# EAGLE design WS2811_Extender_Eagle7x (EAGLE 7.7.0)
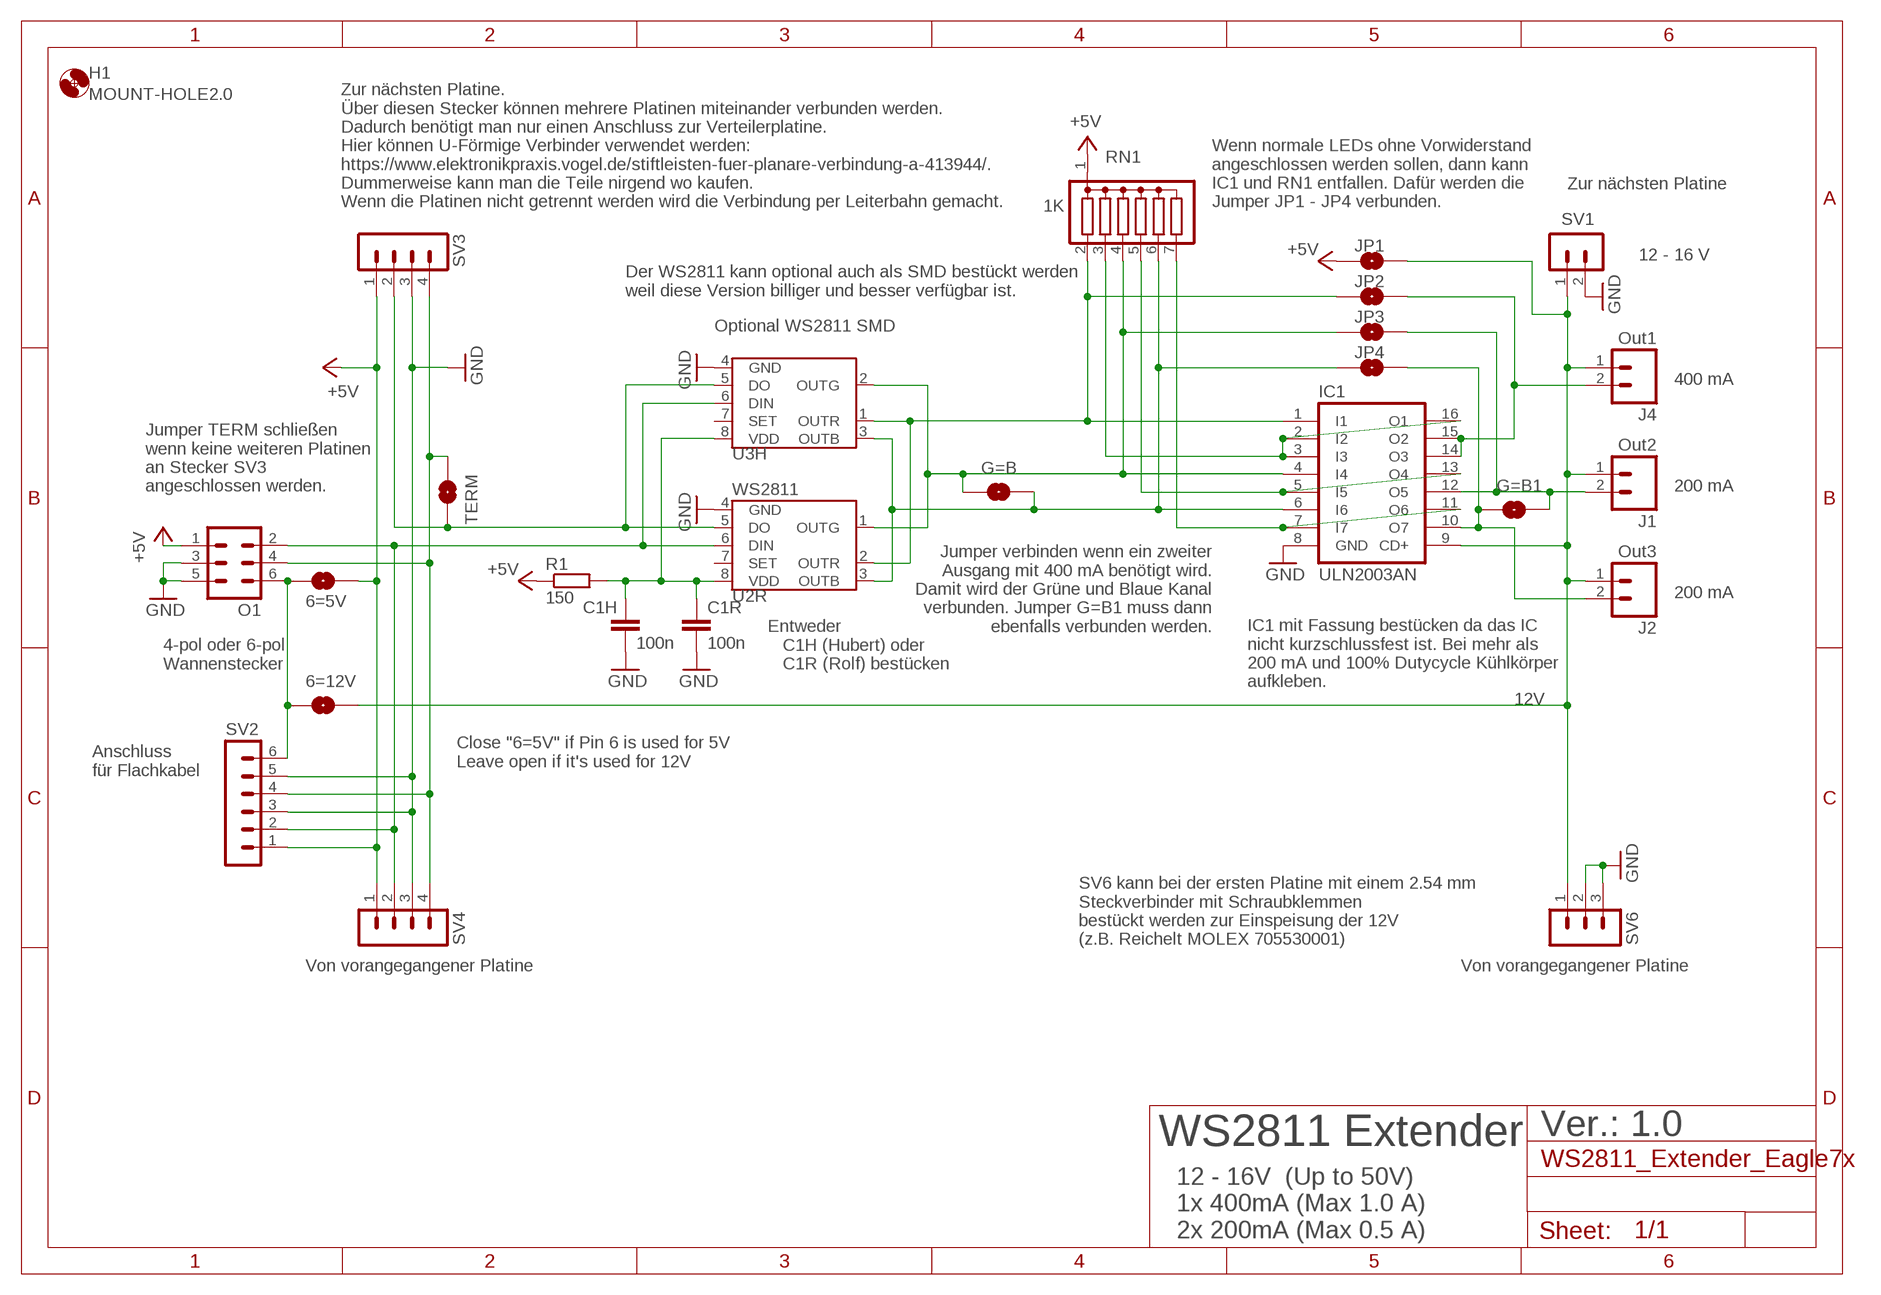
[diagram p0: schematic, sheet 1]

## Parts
6=5V  SOLDERJUMPERNO  [SJ_2S-NO]
6=12V  SOLDERJUMPERNO  [SJ_2S-NO]
C1H  100n  C-EUC1206  [C1206]
C1R  100n  C-EU025-024X044  [C025-024X044]
G=B  SOLDERJUMPERNO  [SJ_2S-NO]
G=B1  SOLDERJUMPERNO  [SJ_2S-NO]
H1  MOUNT-HOLE2.0  [2,0]
IC1  ULN2003AN  [DIL16]
J1  Out2  M02PTH  [1X02]
J2  Out3  M02PTH  [1X02]
J4  Out1  M02PTH  [1X02]
JP1  SOLDERJUMPERNO  [SJ_2S-NO]
JP2  SOLDERJUMPERNO  [SJ_2S-NO]
JP3  SOLDERJUMPERNO  [SJ_2S-NO]
JP4  SOLDERJUMPERNO  [SJ_2S-NO]
O1  ML6  [ML6]
R1  150  RCL_R-EU_0207/2V  [RCL_0207/2V]
RN1  1K  G06R  [SIL7]
SV1  MA02-1  [MA02-1]
SV2  MA06-1  [MA06-1]
SV3  MA04-1  [MA04-1]
SV4  MA04-1  [MA04-1]
SV6  MA03-1  [MA03-1]
TERM  SOLDERJUMPERNO  [SJ_2S-NO]
U2R  WS2811  S3PO_MODUL_WS2811_SOUND_MP3-TF-16P_WS2811_AND_ATTINY_WS2811-ICTINY45-20-DIP  [S3PO_MODUL_WS2811_SOUND_MP3-TF-16P_WS2811_AND_ATTINY_WS2811_DIP08]
U3H  WS2811 SOT-8  S3PO_MODUL_WS2811_SOUND_MP3-TF-16P_WS2811_AND_ATTINY_WS2811-ICSOP8  [SOP8]

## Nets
12V: 6=12V.2 IC1.9(CD+) J1.1 J2.1 J4.1 JP1.2 SV1.1 SV6.1
+5V: 6=5V.2 JP1.1 O1.1 R1.1 RN1.1 SV2.1 SV3.1 SV4.1
GND: C1H.2 C1R.2 IC1.8(GND) O1.3 O1.5 SV1.2 SV2.3 SV2.5 SV3.3 SV4.3 SV6.2 SV6.3 U2R.4(GND) U3H.4(GND)
N$1: O1.2 SV2.2 SV4.2 U2R.6(DIN) U3H.6(DIN)
N$2: SV3.2 TERM.2 U2R.5(DO) U3H.5(DO)
N$3: O1.4 SV2.4 SV3.4 SV4.4 TERM.1
N$4: C1H.1 C1R.1 R1.2 U2R.8(VDD) U3H.8(VDD)
N$5: IC1.1(I1) JP2.1 RN1.2 U2R.2(OUTR) U3H.1(OUTR)
N$6: 6=5V.1 6=12V.1 O1.6 SV2.6
N$8: G=B.2 IC1.6(I6) JP4.1 RN1.6 U2R.3(OUTB) U3H.3(OUTB)
N$9: IC1.2(I2) IC1.3(I3) IC1.16(O1) RN1.3
N$11: IC1.5(I5) IC1.13(O4) RN1.5
N$12: IC1.7(I7) IC1.11(O6) RN1.7
N$21: G=B.1 IC1.4(I4) JP3.1 RN1.4 U2R.1(OUTG) U3H.2(OUTG)
O1: IC1.14(O3) IC1.15(O2) J4.2 JP2.2
O2: G=B1.2 IC1.12(O5) J1.2 JP3.2
O3: G=B1.1 IC1.10(O7) J2.2 JP4.2
Unconnected: U2R.7(SET) U3H.7(SET)

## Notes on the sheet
- Zur nächsten Platine
- Zur nächsten Platine. 
  Über diesen Stecker können mehrere Platinen miteinander verbunden werden.
  Dadurch benötigt man nur einen Anschluss zur Verteilerplatine.
  Hier können U-Förmige Verbinder verwendet werden: 
  https://www.elektronikpraxis.vogel.de/stiftleisten-fuer-planare-verbindung-a-413944/.
  Dummerweise kann man die Teile nirgend wo kaufen.
  Wenn die Platinen nicht getrennt werden wird die Verbindung per Leiterbahn gemacht.
- Wenn normale LEDs ohne Vorwiderstand
  angeschlossen werden sollen, dann kann
  IC1 und RN1 entfallen. Dafür werden die
  Jumper JP1 - JP4 verbunden.
- 12 - 16 V
- Der WS2811 kann optional auch als SMD bestückt werden
  weil diese Version billiger und besser verfügbar ist.
- Optional WS2811 SMD
- 400 mA
- Jumper TERM schließen 
  wenn keine weiteren Platinen
  an Stecker SV3 
  angeschlossen werden.
- 200 mA
- Jumper verbinden wenn ein zweiter
  Ausgang mit 400 mA benötigt wird.
  Damit wird der Grüne und Blaue Kanal
  verbunden. Jumper G=B1 muss dann
  ebenfalls verbunden werden.
- 200 mA
- 4-pol oder 6-pol 
  Wannenstecker
- Entweder 
     C1H (Hubert) oder 
     C1R (Rolf) bestücken
- IC1 mit Fassung bestücken da das IC
  nicht kurzschlussfest ist. Bei mehr als 
  200 mA und 100% Dutycycle Kühlkörper
  aufkleben.
- Close "6=5V" if Pin 6 is used for 5V
  Leave open if it's used for 12V
- Anschluss
  für Flachkabel
- SV6 kann bei der ersten Platine mit einem 2.54 mm
  Steckverbinder mit Schraubklemmen
  bestückt werden zur Einspeisung der 12V
  (z.B. Reichelt MOLEX 705530001)
- Von vorangegangener Platine | Von vorangegangener Platine
- WS2811 Extender | Ver.: 1.0
- 12 - 16V  (Up to 50V)
  1x 400mA (Max 1.0 A)
  2x 200mA (Max 0.5 A)

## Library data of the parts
6=5V 6=12V G=B G=B1 JP1-JP4 TERM = SparkFun-Retired:SOLDERJUMPER: Solder Jumper
C1H C1R = rcl:C-EU: CAPACITOR, European symbol; SPICEPREFIX: C
H1 = holes:MOUNT-HOLE: MOUNTING HOLE with drill center marker
IC1 = uln-udn:ULN2003A: DRIVER ARRAY; REICHELT: ULN 2003A STM; REICHELT_EU: 0,22 €; REICHELT_LNK: https://www.reichelt.de/seven-darlington-arrays-dip-16-uln-2003a-stm-p216685.html?&trstct=pos_0
J1 J2 J4 = SparkFun-Connectors:M02: Standard 2-pin 0.1" header. Use with
O1 = con-harting-ml:ML6: HARTING; OC_FARNELL: unknown; OC_NEWARK: unknown
R1 = Sound_MP3-TF-16P_and_WS2811:RCL_R-EU_: RESISTOR, European symbol; SPICEPREFIX: R
RN1 = resistor-sil:G06R: SIL RESISTOR; OC_FARNELL: unknown; OC_NEWARK: unknown; REICHELT: SIL 7-6 1,0K; REICHELT_EU: 0,071 €; REICHELT_LNK: https://www.reichelt.de/widerstandsnetzwerk-1-0-kohm-sternschaltung-6wid-7pins-sil-7-6-1-0k-p17841.html?&trstct=pol_1
SV1 = con-lstb:MA02-1: PIN HEADER
SV2 = con-lstb:MA06-1: PIN HEADER; OC_FARNELL: unknown; OC_NEWARK: unknown
SV3 SV4 = con-lstb:MA04-1: PIN HEADER
SV6 = con-lstb:MA03-1: PIN HEADER
U2R = S3PO_Modul_WS2811:S3PO_MODUL_WS2811_SOUND_MP3-TF-16P_WS2811_AND_ATTINY_WS2811-IC: Die Pin nummern im Dokument https://cdn-shop.adafruit.com/datasheets/WS2811.pdf für R und G sind vertauscht ;-(; PROD_ID: IC-09439; VALUE: TINY45-20-DIP
U3H = S3PO_Modul_WS2811:S3PO_MODUL_WS2811_SOUND_MP3-TF-16P_WS2811_AND_ATTINY_WS2811-IC: Die Pin nummern im Dokument https://cdn-shop.adafruit.com/datasheets/WS2811.pdf für R und G sind vertauscht ;-(

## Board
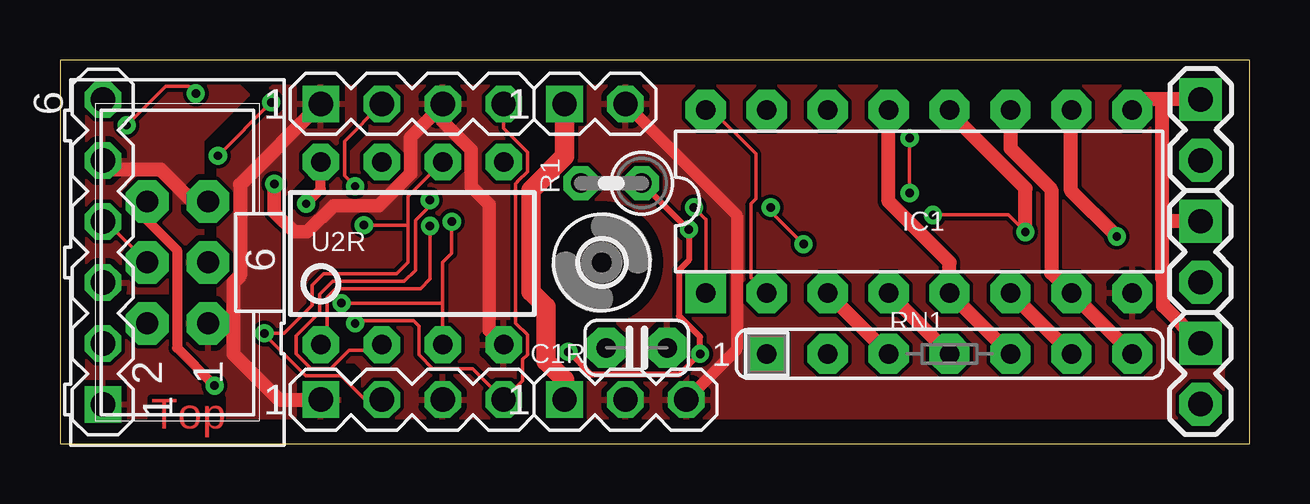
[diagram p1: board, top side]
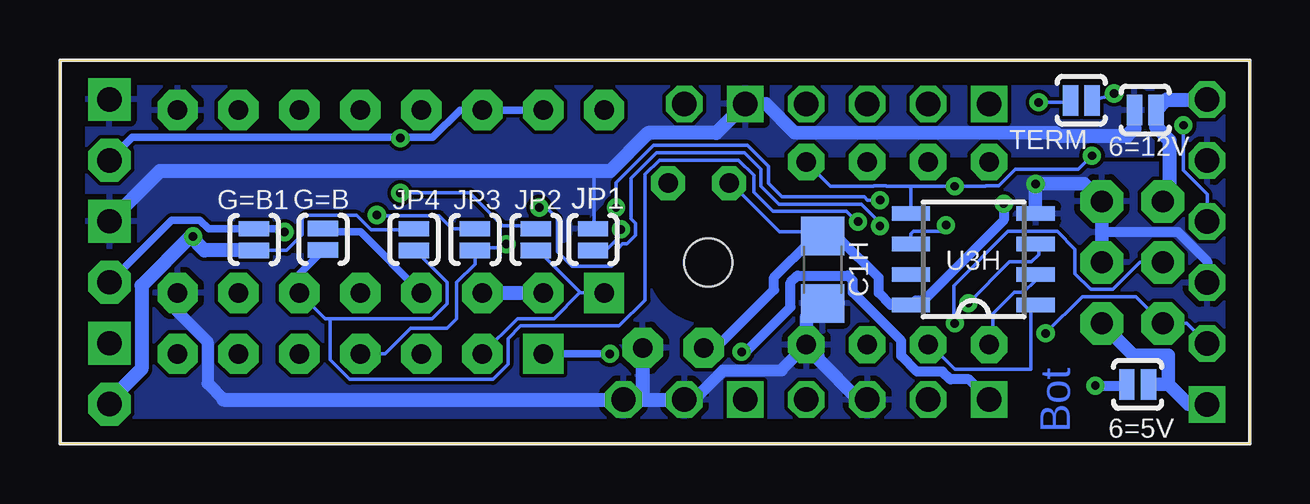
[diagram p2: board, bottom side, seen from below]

Size 49.6 x 15.99 mm. Coordinates in mm from the lower left corner, seen from the top.
Outline: 0,0 49.6,0 49.6,15.99 0,15.99 0,0
Copper layers (1*16): Top 0.035mm / dielectric 1.5mm / Bottom 0.035mm
Design rules "default": minimum track width 6mil, minimum drill 0.35mm, track to track 6mil, track to pad 6mil, pad to pad 6mil, via to via 6mil, smd to smd 6mil, copper to edge 40mil, drill to drill 6mil, minimum pad ring 10mil, minimum via ring 8mil, stop-mask expansion 4mil, vias tented up to drill 0mil, thermal gap 10mil

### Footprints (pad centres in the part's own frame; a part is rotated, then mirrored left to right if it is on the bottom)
SJ_2S-NO = smd 0.635 x 1.27: 1 -0.45,0; 2 0.45,0
C1206 = smd 1.6 x 1.8: 1 -1.4,0; 2 1.4,0
C025-024X044 = drill 0.813 pad 1.676 octagon: 1 -1.27,0; 2 1.27,0
2,0 = hole 2: 0,0
DIL16 = drill 0.813 pad 1.676 square: 1 -8.89,-3.81 | drill 0.813 pad 1.676 octagon: 2 -6.35,-3.81; 3 -3.81,-3.81; 4 -1.27,-3.81; 5 1.27,-3.81; 6 3.81,-3.81; 7 6.35,-3.81; 8 8.89,-3.81; 9 8.89,3.81; 10 6.35,3.81; 11 3.81,3.81; 12 1.27,3.81; 13 -1.27,3.81; 14 -3.81,3.81; 15 -6.35,3.81; 16 -8.89,3.81
1X02 = drill 1.016 pad 1.778 square: 1 0,0 | drill 1.016 pad 1.778 octagon: 2 2.54,0
ML6 = drill 0.914 pad 1.778 octagon: 1 -2.54,-1.27; 2 -2.54,1.27; 3 0,-1.27; 4 0,1.27; 5 2.54,-1.27; 6 2.54,1.27
RCL_0207/2V = drill 0.813 pad 1.422 octagon: 1 -1.27,0; 2 1.27,0
SIL7 = drill 0.813 pad 1.676 square: 1 -7.62,0 | drill 0.813 pad 1.676 octagon: 2 -5.08,0; 3 -2.54,0; 4 0,0; 5 2.54,0; 6 5.08,0; 7 7.62,0
MA02-1 = drill 1.016 pad 1.524 square: 1 -1.27,0 | drill 1.016 pad 1.524 octagon: 2 1.27,0
MA06-1 = drill 1.016 pad 1.524 square: 1 -6.35,0 | drill 1.016 pad 1.524 octagon: 2 -3.81,0; 3 -1.27,0; 4 1.27,0; 5 3.81,0; 6 6.35,0
MA04-1 = drill 1.016 pad 1.524 square: 1 -3.81,0 | drill 1.016 pad 1.524 octagon: 2 -1.27,0; 3 1.27,0; 4 3.81,0
MA03-1 = drill 1.016 pad 1.524 square: 1 -3.81,0 | drill 1.016 pad 1.524 octagon: 2 -1.27,0; 3 1.27,0
S3PO_MODUL_WS2811_SOUND_MP3-TF-16P_WS2811_AND_ATTINY_WS2811_DIP08 = drill 0.813 pad 1.524 octagon: 1 -3.81,-3.81; 2 -1.27,-3.81; 3 1.27,-3.81; 4 3.81,-3.81; 5 3.81,3.81; 6 1.27,3.81; 7 -1.27,3.81; 8 -3.81,3.81
SOP8 = smd 0.6 x 1.6: 1 -1.905,-2.6; 2 -0.635,-2.6; 3 0.635,-2.6; 4 1.905,-2.6; 5 1.905,2.6; 6 0.635,2.6; 7 -0.635,2.6; 8 -1.905,2.6

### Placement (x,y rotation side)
6=5V  4.68,2.48 0 bottom
6=12V  4.36,13.91 180 bottom
C1H  17.81,7.25 270 bottom
C1R  24.04,4 0 top
G=B  38.63,8.52 270 bottom
G=B1  41.51,8.51 90 bottom
H1  22.59,7.55 0 top
IC1  35.81,10.1 0 top
J1  47.54,9.27 270 top
J2  47.54,4.19 270 top
J4  47.54,14.35 270 top
JP1  27.38,8.51 90 bottom
JP2  29.76,8.51 90 bottom
JP3  32.3,8.51 90 bottom
JP4  34.84,8.51 90 bottom
O1  4.9,7.55 90 top
R1  22.98,10.86 180 top
RN1  37.08,3.75 0 top
SV1  22.3,14.16 0 top
SV2  1.78,7.99 90 top
SV3  14.68,14.16 0 top
SV4  14.68,1.84 0 top
SV6  24.84,1.84 0 top
TERM  7.03,14.31 180 bottom
U2R  14.68,7.94 0 top
U3H  11.53,7.68 90 bottom

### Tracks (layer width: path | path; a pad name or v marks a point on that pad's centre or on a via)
12V
  Top 0.584: 45.95,14.35 45.14,14.35 IC1.9 | 45.95,9.46 45.95,6.84 45.98,6.82 45.98,5.74 J2.1 | 45.95,9.46 45.95,14.35 | 45.95,9.46 46.15,9.27 J1.1 | J4.1 45.95,14.35
  Top 0.813: SV1.1 21.03,11.97 19.63,10.57 19.63,6.33 20.25,5.71 20.25,3.44 21.03,2.67 SV6.1
  Bottom 0.152: 27.34,11.37 27.34,9.01 JP1.2
  Bottom 0.559: 20.18,14.16 18.99,12.97 8.12,12.97 8.11,12.95
  Bottom 0.584: 6=12V.2 4.81,13.14 5.12,12.83 7.98,12.83 8.11,12.95 | 20.18,14.16 SV1.1 22.24,12.95 25.08,12.95 26.67,11.37 27.34,11.37 45.44,11.37 J1.1
  pour Bottom: 48.5,15.18 4.36,15.18 4.04,14.86 4.04,12 25,12 28.81,8.19 48.5,8.19
+5V  (via drill 0.35)
  Top 0.254: v21.19,3.83 22.14,2.88 25.82,2.88 v26.68,3.75 26.68,4.45 25.8,5.33 25.8,7.24 26.22,7.65 v26.22,8.93 26.18,8.93 R1.1
  Top 0.584: 7.22,5.01 7.22,6.72 7.51,7 7.51,10.79 SV3.1 | 7.22,5.01 7.22,3.75 9.12,1.84 SV4.1 | O1.1 7.22,5.01
  Bottom 0.152: v26.22,8.93 26.36,8.79 26.36,8.54 26.85,8.06 JP1.1
  Bottom 0.305: RN1.1 v26.68,3.75
  Bottom 0.406: v21.19,3.83 21,3.83 19.14,5.69 19.14,6.72 18.86,7.01 16.77,7.01 16.56,6.8 16.56,6.31 14.53,4.28 14.53,3.66 13.87,3.01 12.81,3.01 12.48,2.68 11.71,2.68 SV4.1
  Bottom 0.559: O1.1 4.85,3.69 3.41,3.69 3.41,2.48 | 6=5V.2 3.41,2.48 | 3.41,2.48 2.57,1.64 SV2.1
  pour Top: 12.3,15.18 12.3,13.27 9.12,10.1 9.12,3.75 10.08,2.79 11.66,2.79 11.66,0.25 0.23,0.25 0.23,4.7 1.19,5.65 6.27,5.65 6.58,5.97 6.58,12 8.49,13.91 8.49,14.54 9.12,15.18
GND  (via drill 0.35)
  Top 0.152: 15.88,14.05 SV3.3
  Top 0.508: SV1.2 28.21,9.52 28.21,3.94 SV6.3
  Top 0.559: 15.88,14.05 14.61,12.77 14.61,11.25 13.27,9.92 11.41,9.92 10.31,8.83 9.76,8.83 8.94,9.65 v8.94,10.83 | U2R.4 17.89,4.73 17.89,9.99 17.15,10.73 17.15,12.24 15.95,13.43 SV3.3
  Top 0.584: SV2.5 2.15,11.43 4.18,11.43 5.52,10.1 O1.5
  Bottom 0.406: 6.17,8.83 3,8.83 1.78,7.6 SV2.3
  Bottom 0.508: U2R.4 19.51,3.1 19.51,3.05 21.96,3.05 23.17,1.84 | IC1.8 44.7,5.5 43.45,4.26 43.45,2.51 42.78,1.84
  Bottom 0.559: O1.3 6.17,8.83 O1.5 6.9,10.83 v8.94,10.83 U3H.4 | C1H.2 18.49,5.27 U2R.4 18.01,3.64 18.01,3.54 16.31,1.84 SV4.3
  Bottom 0.584: 42.78,1.84 SV6.3 25.32,1.84 | 25.32,1.84 SV6.2 23.17,1.84 | C1R.2 25.31,1.85 25.32,1.84
  pour Bottom: 48.5,0.57 0.55,0.57 0.55,15.18 3.09,15.18 3.09,12.32 3.73,11.68 24.68,11.68 28.49,7.87 48.5,7.87
  pour Top: 0.87,6.28 5.95,6.28 5.95,11.37 5.95,12.63 7.86,14.54 7.22,15.18 0.23,15.18 0.23,6.92
  pour Top: 12.62,0.57 48.5,0.57 49.13,1.21 49.13,15.18 13.25,15.18 12.94,14.86 12.94,12.95 9.76,9.78 9.76,9.14 9.76,4.38 10.08,4.06 10.71,3.43 12.3,3.43 12.62,3.11 12.62,2.79
N$1  (via drill 0.35)
  Top 0.152: SV4.2 12.72,1.84 11.73,2.83 10.24,2.83 8.52,4.56 v8.52,4.6 9.35,4.6 10.52,5.77 10.52,6.6 10.99,7.08 14.03,7.08 14.51,7.55 14.51,9.14 | 14.51,9.14 14.51,10.31 U2R.6 | v12.67,9.11 14.48,9.11 14.51,9.14
  Bottom 0.152: v8.52,4.6 6.99,6.13 4.76,6.13 3.65,5.01 O1.2 2.62,5.01 SV2.2 | v12.67,9.11 12.93,8.85 14.03,8.85 14.13,8.75 U3H.6
N$2  (via drill 0.35)
  Top 0.152: v8.81,14.22 v6.58,12 | v12.3,10.73 11.86,11.17 11.86,12.61 SV3.2
  Bottom 0.152: v8.81,14.22 7.8,14.22 TERM.2 | 14.21,10.73 v12.3,10.73 11.03,10.73 11,10.76 10.46,10.76 9.78,11.43 7.15,11.43 v6.58,12 | 14.21,10.73 15.14,10.73 15.17,10.76 15.67,10.76 15.7,10.73 17.48,10.73 U2R.5 | U3H.5 14.13,10.66 14.21,10.73
N$3  (via drill 0.35)
  Top 0.152: SV3.4 18.49,13.15 19.48,12.16 19.48,11.34 19.08,10.93 19.08,10.92 19,10.84 19,5.02 19.48,4.54 19.48,3.72 19.29,3.52 19.29,2.63 SV4.4 17.2,3.14 15.54,3.14 14.96,3.72 14.96,4.89 14.74,5.12 12.4,5.12 v12.3,5.01 | O1.4 1.93,9.26 SV2.4 | v2.77,13.27 4.4,14.9 5.36,14.9 v5.66,14.6
  Bottom 0.152: TERM.1 5.66,14.54 v5.66,14.6 | O1.4 4.59,7.55 5.71,6.44 6.63,6.44 7.29,7.09 7.29,8.1 8.04,8.85 10.09,8.85 12.34,6.59 12.34,5.06 v12.3,5.01 | SV2.4 1.78,10.4 2.77,11.39 v2.77,13.27
N$4  (via drill 0.35)
  Top 0.406: v10.26,10 10.87,10.61 U2R.8
  Bottom 0.152: C1H.1 17.99,8.83 19.6,8.83 21.64,10.86 R1.2
  Bottom 0.203: 17.81,8.51 C1H.1
  Bottom 0.406: v10.26,10 10.26,9.31 13.57,6 13.57,5.97 13.94,5.97 U3H.8 14.97,5.78 15.47,6.28 15.47,6.92 17.06,8.51 17.81,8.51 18.26,8.51 19.83,6.94 19.83,6.42 22.25,4 C1R.1
N$5  (via drill 0.35)
  Top 0.152: U2R.2 13.19,3.9 12.05,3.9 11.28,3.14 10.46,3.14 9.85,3.75 9.85,4.51 10.82,5.48 10.82,6.24 11.36,6.77 14.35,6.77 14.82,7.23 14.82,9.32 15.42,9.93 v15.42,10.15 | IC1.1 26.92,9.35 26.88,9.38 v26.42,9.84
  Bottom 0.152: U3H.1 9.12,5.65 9.12,3.11 12.3,3.11 13.25,4.06 U2R.2 | v15.42,10.15 15.94,10.15 16.08,10.29 19.51,10.29 20.07,10.86 20.07,11.57 20.94,12.43 24.87,12.43 26.42,10.88 v26.42,9.84 | RN1.2 30.52,5.22 29.02,5.22 27.95,6.28 | 27.95,6.28 IC1.1 | JP2.1 29.62,8.01 27.95,6.34 27.95,6.28
N$6  (via drill 0.35)
  Top 0.406: O1.6 3.63,9.32 4.88,8.07 4.88,3.99 v6.44,2.42
  Bottom 0.406: v6.44,2.42 5.18,2.42 6=5V.1
  Bottom 0.584: O1.6 3.35,10.38 3.35,12.63 3.91,13.2 6=12V.1 3.48,14.34 SV2.6
N$8  (via drill 0.35)
  Top 0.152: v11.73,5.86 15.91,5.86 15.95,5.9 | 15.95,5.9 15.95,7.55 16.33,7.94 v16.33,9.26 | 15.95,5.9 U2R.3
  Top 0.584: IC1.6 RN1.6
  Bottom 0.152: v16.33,9.26 16.4,9.26 16.82,9.68 19.89,9.68 20.68,10.48 20.68,11.19 21.32,11.82 24.61,11.82 25.21,11.22 25.21,5.99 26.29,4.91 30.4,4.91 30.93,4.38 30.93,3.3 31.56,2.68 37.52,2.68 38.34,3.49 38.34,5.22 | U3H.3 8.81,8.19 8.81,7.87 9.1,7.58 10.02,7.58 v11.73,5.86 | JP4.1 34.8,8.06 33.47,6.73 33.47,5.84 34.1,5.22 38.34,5.22 | IC1.6 38.55,5.22 38.34,5.22
  Bottom 0.305: G=B.2 39.62,7.09 IC1.6
N$9
  Top 0.152: IC1.2 28.82,6.92 28.81,6.92 28.81,10 29.01,10.2 29.01,12.07 27.18,13.91 IC1.16
  Top 0.584: IC1.3 RN1.3
  Bottom 0.584: IC1.3 IC1.2
N$11
  Top 0.584: RN1.5 IC1.5 37.08,7.55 34.54,10.1 IC1.13
N$12
  Top 0.584: RN1.7 IC1.7 41.32,7.12 41.32,10.6 39.62,12.3 IC1.11
N$21  (via drill 0.35)
  Top 0.152: v15.42,9.07 15.42,6.87 15.02,6.47 11.48,6.47 11.13,6.11 11.13,4.38 U2R.1 | v30.99,8.32 29.62,9.69 v29.62,9.84
  Top 0.584: IC1.4 RN1.4
  Bottom 0.152: U2R.1 10.71,4.38 10.71,5.42 9.83,6.31 9.44,6.31 8.93,6.82 U3H.2 | v15.42,9.07 15.42,9.21 16.2,9.98 19.63,9.98 20.38,10.73 20.38,11.44 21.06,12.13 24.74,12.13 25.81,11.06 25.81,9.38 25.61,9.18 25.61,8.68 25.96,8.33 26.15,8.33 26.36,8.11 26.36,7.64 26.6,7.4 28.26,7.4 28.86,8 28.86,9.38 29.32,9.84 v29.62,9.84 | RN1.4 36.05,3.75 34.98,4.81 33.46,4.81 33.07,5.21 33.07,6.73 32.3,7.49 JP3.1 32.21,8.17 31.15,8.17 v30.99,8.32
  Bottom 0.305: G=B.1 38.49,8.83 37.08,8.83 IC1.4
O1  (via drill 0.35)
  Top 0.152: v35.41,12.74 v35.41,10.45
  Bottom 0.152: v35.41,10.45 32.52,10.45 31.15,9.08 29.78,9.08 JP2.2 | v35.41,12.74 35.41,12.76
  Bottom 0.305: J4.2 46.59,12.76 35.41,12.76 34.06,12.76 32.92,13.91 IC1.14 IC1.15
O2  (via drill 0.35)
  Top 0.152: v36.39,9.53 39.53,9.53 v40.24,8.83
  Top 0.584: v40.24,8.83 40.24,10.64 37.08,13.8 IC1.12
  Bottom 0.152: JP3.2 33.25,8.96 33.8,9.5 36.36,9.5 v36.39,9.53
  Bottom 0.305: v40.24,8.83 40.37,8.96 G=B1.2 43.4,8.96 43.77,9.32 44.95,9.32 J1.2
O3  (via drill 0.35)
  Top 0.584: IC1.10 42.15,13.89 42.15,10.54 v44.05,8.64
  Bottom 0.152: JP4.2 34.98,8.93 36.64,8.93 37.23,9.52 39.36,9.52 39.5,9.38 39.5,8.71 40.15,8.06 G=B1.1
  Bottom 0.584: J2.2 47.54,1.78 46.2,3.12 46.2,6.59 44.16,8.64 | v44.05,8.64 44.16,8.64 | G=B1.1 43.58,8.06 44.16,8.64

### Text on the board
Top: Top
Bottom: Bot
tDocu: + | Out 1 | + | Out 2 | + | Out 3 | WS2811 Extender V 1.0
bDocu: 5/12V | => | <= | +5V | GND | +12V | GND | + | Out 1 | GND | max 50V | 400 mA | WS2811 Extender | Out | + | Out 2 | GND | 200 mA | In | + | Out 3 | 1 | 200 mA | +5V | <= | +5V | => | GND | +12V | GND | Stummis & Hardi | 29.10.19

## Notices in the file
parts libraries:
SparkFun-Retired: Licensing:Creative Commons ShareAlike 4.0 International - https://creativecommons.org/licenses/by-sa/4.0
